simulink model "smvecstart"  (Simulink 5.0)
settings: Solver=ode45  StartTime=0.0  StopTime=12  MaxStep=1e-3  RelTol=1e-4  AbsTol=1e-4
InitFcn:
  | smvecstartdef
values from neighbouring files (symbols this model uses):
  Bm = 0.10    (= 0.1)    [IMabc2.m]    (also in imabcparam.m = 0.01; IMabcrun0.m = 0.01; IMabcrun1.m = 0.001; IMcur0.m = 1e-06)
  H = 0.60    (= 0.6)    [IMabc2.m]    (also in IMcur0.m = 0.3; imdef0vec.m = 0.3; imdef1vec.m = 0.3; imdef2vec.m = 0.3)
  Ra = .95    (= 0.95)    [altwdgs.m]    (also in Ccurverun.m = 0.018)
  V = [Vas 0 0].'    [Actac.m]    (also in acttrcalc1.m = str2num(get(h,'string')); im3d.m = eval(get(hVs,'String')); IMabc2.m = [vas vbs vcs 0 0 0]'; IMabcf0.m = [vas vbs vcs 0 0 0]')
  wo = 2*pi*freq0    [calc0.m]    (also in IMabc2.m = 376.991118431; imabcparam.m = 376.991118431; IMabcrun0.m = 376.991118431; IMabcrun1.m = 376.991118431)
undefined symbols (not defined in the file or in its folder): L_1, Rf, Rfstart, Rkd, Rkq
libraries: simulink x1

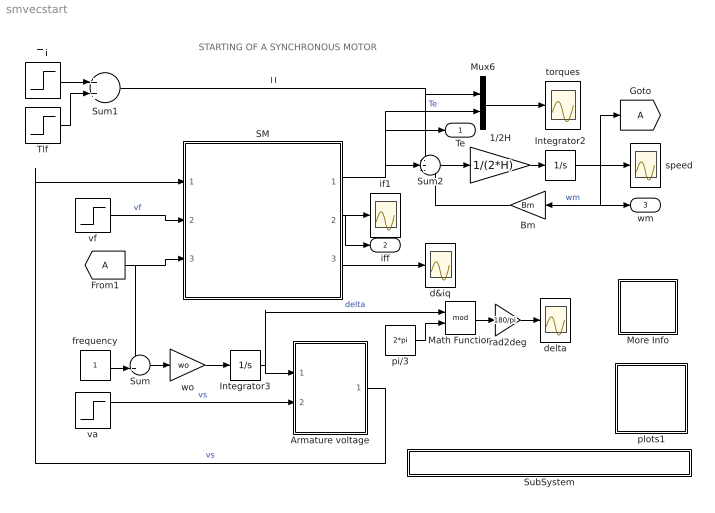
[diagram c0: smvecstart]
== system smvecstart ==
  note: STARTING OF A SYNCHRONOUS MOTOR
  1/2H : Gain  Gain=1/(2*H)
  Armature voltage : Subsystem
  Bm : Gain  Orientation=left  Gain=Bm
  Integrator2 : Integrator
  Integrator3 : Integrator
  Math Function : Math  Operator=mod
  More Info : Subsystem
  Mux6 : Mux  Inputs=2
  SM : Subsystem
  SubSystem : Subsystem
  Sum : Sum  Inputs=-+|
  Sum1 : Sum
  Sum2 : Sum  Inputs=-+-
  Tlf : Step  Time=10  Before=0.0  After=0.8  SampleTime=0
  Tli : Step  Time=0  After=0.2  SampleTime=0
  d&iq : Scope
  delta : Scope
  frequency : Constant
  if1 : Scope
  pi/3 : Constant  Value=2*pi
  plots1 : Subsystem
  rad2deg : Gain  Gain=180/pi
  speed : Scope
  torques : Scope
  va : Step  Time=0  After=V  SampleTime=0
  vf : Step  Time=5  After=0.02  SampleTime=0
  wo : Gain  Gain=wo
  Te : Outport
  iff : Outport  Port=2
  wm : Outport  Port=3
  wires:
  Mux6/1 -> torques/1
  vf/1 -> SM/2(vf)  "vf"
  [A] -> SM/3(wm), Sum/1
  Sum2/1 -> 1/2H/1
  1/2H/1 -> Integrator2/1
  SM/1(Te) -> Sum2/2, Mux6/2, Te/1  "Te"
  Bm/1 -> Sum2/3
  Integrator2/1 -> speed/1, [A], Bm/1, wm/1  "wm"
  Armature voltage/1(vs) -> SM/1(vs)  "vs"
  SM/3(ia) -> d&iq/1
  va/1 -> Armature voltage/2(Vt)  "vs"
  Tli/1 -> Sum1/1
  Tlf/1 -> Sum1/2
  Sum1/1 -> Mux6/1, Sum2/1  "Tl"
  Integrator3/1 -> Armature voltage/1(delta), Math Function/1  "delta"
  frequency/1 -> Sum/2
  Sum/1 -> wo/1
  wo/1 -> Integrator3/1
  SM/2(if) -> if1/1, iff/1
  Math Function/1 -> rad2deg/1
  pi/3/1 -> Math Function/2
  rad2deg/1 -> delta/1

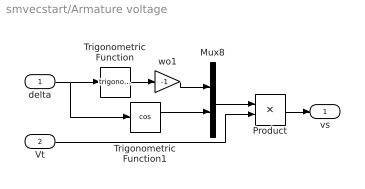
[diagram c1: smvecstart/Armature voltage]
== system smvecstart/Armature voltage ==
  delta : Inport
  Vt : Inport  Port=2
  Mux8 : Mux  Inputs=2
  Product : Product
  Trigonometric Function : Trigonometry
  Trigonometric Function1 : Trigonometry  Operator=cos
  wo1 : Gain  Gain=-1
  vs : Outport
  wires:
  delta/1 -> Trigonometric Function/1, Trigonometric Function1/1
  Trigonometric Function/1 -> wo1/1
  Mux8/1 -> Product/1
  wo1/1 -> Mux8/1
  Trigonometric Function1/1 -> Mux8/2
  Product/1 -> vs/1
  Vt/1 -> Product/2

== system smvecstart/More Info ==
  note: This demo simulates the STARTING of a synchronous motor

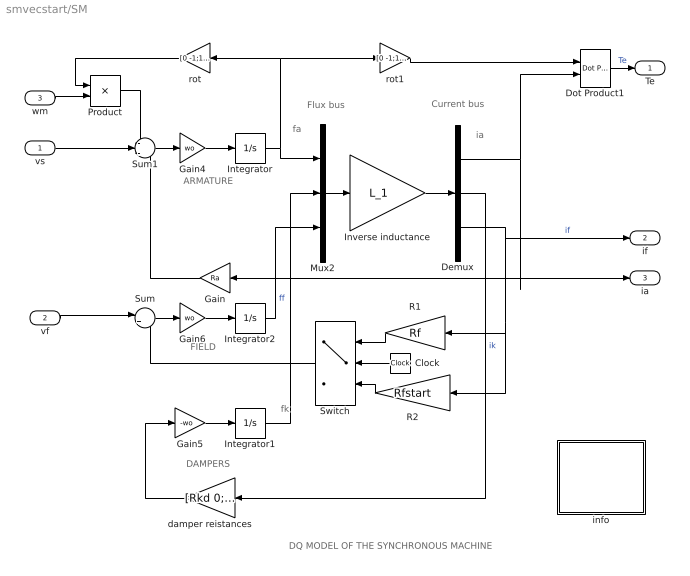
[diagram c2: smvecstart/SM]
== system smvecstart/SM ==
  note: DAMPERS
  note: ARMATURE
  note: fa
  note: fk
  note: ia
  note: FIELD
  note: DQ MODEL OF THE SYNCHRONOUS MACHINE
  note: Flux bus
  note: Current bus
  vs : Inport
  vf : Inport  Port=2
  wm : Inport  Port=3
  Clock : Clock
  Demux : Demux  Outputs=3
  Dot Product1 : simulink/Math Operations/Dot Product
  Gain : Gain  Orientation=left  Gain=Ra
  Gain4 : Gain  Gain=wo
  Gain5 : Gain  Gain=-wo
  Gain6 : Gain  Gain=wo
  Integrator : Integrator  InitialCondition=[0 0]
  Integrator1 : Integrator  InitialCondition=[0 0]
  Integrator2 : Integrator
  Inverse inductance : Gain  Gain=L_1  Multiplication=Matrix(K*u)
  Mux2 : Mux  Inputs=3
  Product : Product
  R1 : Gain  Orientation=left  Gain=Rf
  R2 : Gain  Orientation=left  Gain=Rfstart
  Sum : Sum  Inputs=|+-
  Sum1 : Sum  Inputs=-+-
  Switch : Switch  Orientation=left  Threshold=5
  damper reistances : Gain  Orientation=left  Gain=[Rkd 0;0 Rkq]  Multiplication=Matrix(K*u)
  info : Subsystem
  rot : Gain  Orientation=left  Gain=[0 -1;1 0]  Multiplication=Matrix(K*u)
  rot1 : Gain  Gain=[0 -1;1 0]  Multiplication=Matrix(K*u)
  Te : Outport
  if : Outport  Port=2
  ia : Outport  Port=3
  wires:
  Product/1 -> Sum1/1
  rot/1 -> Product/1
  wm/1 -> Product/2
  Gain5/1 -> Integrator1/1
  damper reistances/1 -> Gain5/1
  Integrator/1 -> Mux2/1, rot/1, rot1/1
  Sum1/1 -> Gain4/1
  Gain4/1 -> Integrator/1
  vs/1 -> Sum1/2
  Gain/1 -> Sum1/3
  Gain6/1 -> Integrator2/1
  Sum/1 -> Gain6/1
  vf/1 -> Sum/1
  rot1/1 -> Dot Product1/1
  Demux/1 -> Gain/1, ia/1, Dot Product1/2
  Dot Product1/1 -> Te/1  "Te"
  Mux2/1 -> Inverse inductance/1
  Inverse inductance/1 -> Demux/1
  R2/1 -> Switch/3
  R1/1 -> Switch/1
  Clock/1 -> Switch/2
  Switch/1 -> Sum/2
  Integrator1/1 -> Mux2/2
  Integrator2/1 -> Mux2/3  "ff"
  Demux/3 -> if/1, R2/1, R1/1  "if"
  Demux/2 -> damper reistances/1  "ik"

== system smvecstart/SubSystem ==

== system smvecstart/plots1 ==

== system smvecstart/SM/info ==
  note: This demonstration illustrates the dynamics of a synchronous generator, initially at no load, following a three-phase short circuit at the terminals.
  note: Synchronous machine transients under shortcircuit
